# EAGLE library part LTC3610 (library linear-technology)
12A, 24V Monolithic Synchronous Step-Down DC/DC Converter Source: http://www.linear.com ..
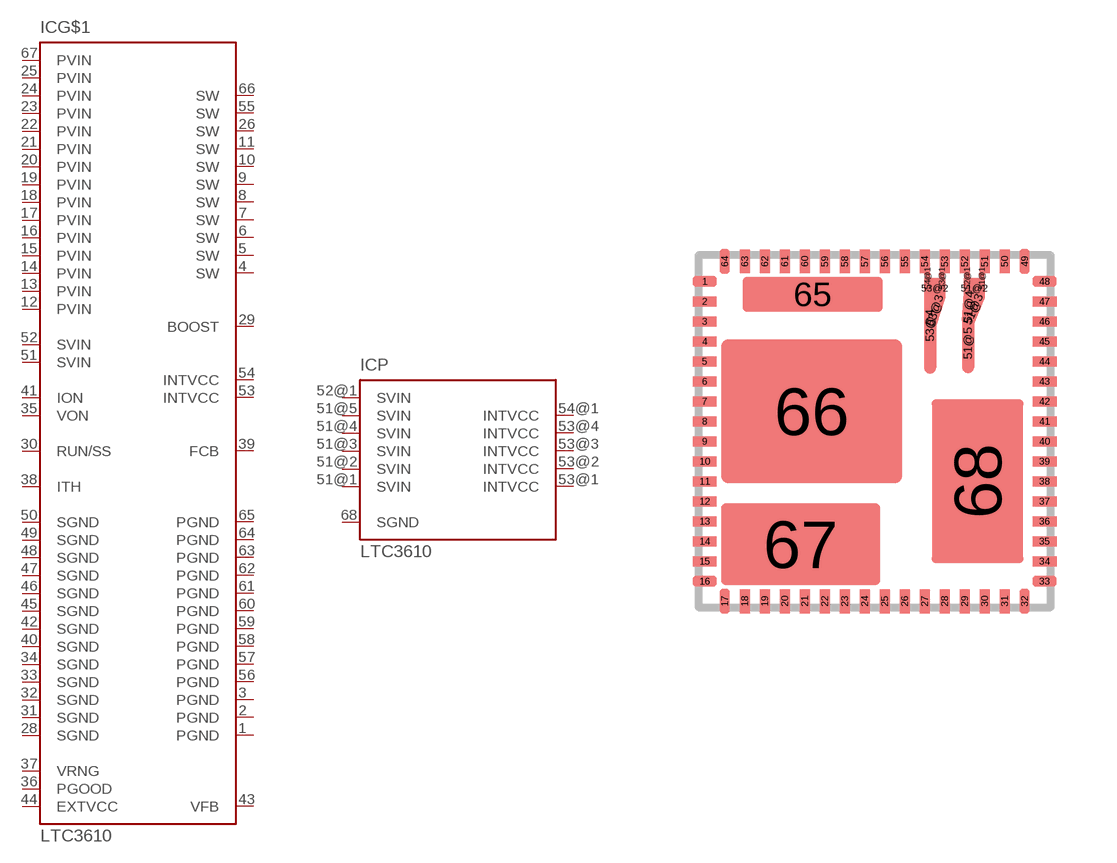
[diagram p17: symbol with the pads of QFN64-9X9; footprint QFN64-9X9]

Designator prefix IC; gates G$1=LTC3610 P=LTC3610-P

## LTC3610 (MPN: LTC3610EWP#PBF; OC_FARNELL: 1536304; OC_NEWARK: 56M8026)  [QFN64-9X9]
1  G$1:PGND  pwr
2  G$1:PGND  pwr
3  G$1:PGND  pwr
4  G$1:SW  in
5  G$1:SW  in
6  G$1:SW  in
7  G$1:SW  in
8  G$1:SW  in
9  G$1:SW  in
10  G$1:SW  in
11  G$1:SW  in
12  G$1:PVIN  pwr
13  G$1:PVIN  pwr
14  G$1:PVIN  pwr
15  G$1:PVIN  pwr
16  G$1:PVIN  pwr
17  G$1:PVIN  pwr
18  G$1:PVIN  pwr
19  G$1:PVIN  pwr
20  G$1:PVIN  pwr
21  G$1:PVIN  pwr
22  G$1:PVIN  pwr
23  G$1:PVIN  pwr
24  G$1:PVIN  pwr
25  G$1:PVIN  pwr
26  G$1:SW  in
28  G$1:SGND  pwr
29  G$1:BOOST  pas
30  G$1:RUN/SS  pas
31  G$1:SGND  pwr
32  G$1:SGND  pwr
33  G$1:SGND  pwr
34  G$1:SGND  pwr
35  G$1:VON  in
36  G$1:PGOOD  oc
37  G$1:VRNG  pas
38  G$1:ITH  pas
39  G$1:FCB  pas
40  G$1:SGND  pwr
41  G$1:ION  in
42  G$1:SGND  pwr
43  G$1:VFB  pas
44  G$1:EXTVCC  in
45  G$1:SGND  pwr
46  G$1:SGND  pwr
47  G$1:SGND  pwr
48  G$1:SGND  pwr
49  G$1:SGND  pwr
50  G$1:SGND  pwr
51  G$1:SVIN  in
51@1  P:SVIN  in
51@2  P:SVIN  in
51@3  P:SVIN  in
51@4  P:SVIN  in
51@5  P:SVIN  in
52  G$1:SVIN  in
52@1  P:SVIN  in
53  G$1:INTVCC  pwr
53@1  P:INTVCC  pwr
53@2  P:INTVCC  pwr
53@3  P:INTVCC  pwr
53@4  P:INTVCC  pwr
54  G$1:INTVCC  pwr
54@1  P:INTVCC  pwr
55  G$1:SW  in
56  G$1:PGND  pwr
57  G$1:PGND  pwr
58  G$1:PGND  pwr
59  G$1:PGND  pwr
60  G$1:PGND  pwr
61  G$1:PGND  pwr
62  G$1:PGND  pwr
63  G$1:PGND  pwr
64  G$1:PGND  pwr
65  G$1:PGND  pwr
66  G$1:SW  in
67  G$1:PVIN  pwr
68  P:SGND  pwr

## Footprint QFN64-9X9 (pad centres in mm)
64-Lead QFN Multipad (9mm × 9mm) Source: http://www.linear.com ..
smd 0.6 x 0.25: 1 -4.25,3.75; 2 -4.25,3.25; 3 -4.25,2.75; 4 -4.25,2.25; 5 -4.25,1.75; 6 -4.25,1.25; 7 -4.25,0.75; 8 -4.25,0.25; 9 -4.25,-0.25; 10 -4.25,-0.75; 11 -4.25,-1.25; 12 -4.25,-1.75; 13 -4.25,-2.25; 14 -4.25,-2.75; 15 -4.25,-3.25; 16 -4.25,-3.75; 33 4.25,-3.75; 34 4.25,-3.25; 35 4.25,-2.75; 36 4.25,-2.25; 37 4.25,-1.75; 38 4.25,-1.25; 39 4.25,-0.75; 40 4.25,-0.25; 41 4.25,0.25; 42 4.25,0.75; 43 4.25,1.25; 44 4.25,1.75; 45 4.25,2.25; 46 4.25,2.75; 47 4.25,3.25; 48 4.25,3.75
smd 0.25 x 0.6: 17 -3.75,-4.25; 18 -3.25,-4.25; 19 -2.75,-4.25; 20 -2.25,-4.25; 21 -1.75,-4.25; 22 -1.25,-4.25; 23 -0.75,-4.25; 24 -0.25,-4.25; 25 0.25,-4.25; 26 0.75,-4.25; 27 1.25,-4.25; 28 1.75,-4.25; 29 2.25,-4.25; 30 2.75,-4.25; 31 3.25,-4.25; 32 3.75,-4.25; 49 3.75,4.25; 50 3.25,4.25; 51 2.75,4.25; 52 2.25,4.25; 53 1.75,4.25; 54 1.25,4.25; 55 0.75,4.25; 56 0.25,4.25; 57 -0.25,4.25; 58 -0.75,4.25; 59 -1.25,4.25; 60 -1.75,4.25; 61 -2.25,4.25; 62 -2.75,4.25; 63 -3.25,4.25; 64 -3.75,4.25
smd 0.16 x 0.3: 51@1 2.68,3.83; 52@1 2.31,3.83; 53@1 1.68,3.83; 54@1 1.32,3.83
smd 0.53 x 0.5: 51@2 2.495,3.58; 53@2 1.505,3.58
smd 0.3 x 1 rotated 157: 51@3 2.475,3.045
smd 0.3 x 1 rotated 176: 51@4 2.36,3.1
smd 0.3 x 1.5: 51@5 2.34,2.195
smd 0.3 x 1 rotated 162: 53@3 1.51,3.015
smd 0.3 x 2.4: 53@4 1.39,2.64
smd 3.5 x 0.87: 65 -1.55,3.425
smd 4.53 x 3.6: 66 -1.575,0.5
smd 3.99 x 2.04: 67 -1.85,-2.825
smd 2.3 x 4.1: 68 2.575,-1.25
